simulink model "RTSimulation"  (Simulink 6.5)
settings: Solver=FixedStepDiscrete  StartTime=0.0  StopTime=inf  RelTol=1e-3
PreLoadFcn:
  | initialize
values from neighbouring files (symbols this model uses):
  actParams = [	bulkModulus   * pressCanon    [Copy of initialize.m]    (also in initialize.m = [bulkModulus	* pressCanon,)
  displFreq = inf    [initialize.m]
  flowCanon = 1.666667e+04    (= 16666.67)    [Copy of initialize.m]    (also in initialize.m)
  forceCanon = 1    [Copy of initialize.m]    (also in initialize.m)
  forceFreq = inf    [initialize.m]
  friction = 5			 				* 0.155000	 				* 0.00444822 				* area1    (= 2.71252900422)    [initialize.m]
  fsamp = 1 / samplePeriod    (= 1024)    [Copy of initialize.m]    (also in initialize.m; rampth.m = 1 / deltaT; randth.m = 1 / deltaT; rspect.m = 1.0 / tsamp)
  gasConstant = 1.8    [Copy of initialize.m]    (also in initialize.m)
  lengthCanon = 1    [Copy of initialize.m]    (also in initialize.m)
  massCanon = 1e-06    [Copy of initialize.m]    (also in initialize.m)
  maxDispl = ( (stroke2 + endLength2) * lengthCanon)'    [Copy of initialize.m]    (also in initialize.m = 576.2)
  maxOilVolume = volume * (1 - (precharge/supplyPress)^(1/gasConstant))    (= 211.391477114)    [Copy of initialize.m]    (also in initialize.m)
  maxVeloc = ( (maxFlow' * flowCanon ./ (area1 * areaCanon)) / velocCanon)'    [Copy of initialize.m]    (also in initialize.m = (maxFlow * flowCanon / (area1 * areaCanon)) / velocCanon; rampth.m = 2 * maxDispl / (nVeloc * deltaT))
  minDispl = (-(stroke1 + endLength1) * lengthCanon)'    [Copy of initialize.m]    (also in initialize.m = -576.2)
  minVeloc = (-(maxFlow' * flowCanon ./ (area2 * areaCanon)) / velocCanon)'    [Copy of initialize.m]    (also in initialize.m = -(maxFlow * flowCanon / (area2 * areaCanon)) / velocCanon)
  nAct = 5    [Copy of initialize.m]    (also in initialize.m = 1)
  nAdcU = 6    [Copy of initialize.m]    (also in initialize.m = 5)
  nDout = 4    [Copy of initialize.m]    (also in initialize.m)
  nDucU = 2    [Copy of initialize.m]    (also in initialize.m)
  nEncU = 3    [Copy of initialize.m]    (also in initialize.m)
  node = completenodestruct(node)    [Copy of initialize.m]    (also in initialize.m)
  precharge = 3000		 				* 6.894757e-03    (= 20.684271)    [Copy of initialize.m]    (also in initialize.m)
  pumpFlow = 1e20    (= 1e+20)    [Copy of initialize.m]    (also in initialize.m)
  returnPress = 3			 				* 0.1    (= 0.3)    [Copy of initialize.m]    (also in initialize.m)
  samplePeriod = controlPeriod/upsampleFactor    (= 0.0009765625)    [Copy of initialize.m]    (also in initialize.m; viewer.m = eval(getHeaderValue(header, 'DELTA_T')))
  springCanon = 1    [Copy of initialize.m]    (also in initialize.m)
  supplyPress = 280		 				* 0.1    (= 28)    [Copy of initialize.m]    (also in initialize.m)
  velocCanon = 1    [Copy of initialize.m]    (also in initialize.m)
  volume = 15.15		 				+ (  45		 				    * 2		 				   + 30		 				    * 6 )	 				* 5    (= 1365.15)    [Copy of initialize.m]    (also in initialize.m; quake.m = volume / 231.0)
  volumeCanon = 1e+06    (= 1000000)    [Copy of initialize.m]    (also in initialize.m)
  yieldDispl = 1.0    (= 1)    [initialize.m]
undefined symbols (not defined in the file or in its folder): DiscIntNeverNeededParam, dpforceFreq, mass, spring, staticForce
libraries: xpclib x5
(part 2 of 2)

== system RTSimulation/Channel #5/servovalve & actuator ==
  note: Parameter vector: 1: oil bulk modulus (force/displ^2) 2: servovalve delay (sec) 3: servovalve overlap 4: rated pressure (force/displ^2) 5: rated flow at rated pressure (displ^3/sec) 6: nominal flow at rated pressure (displ^3/sec) 7: actuator piston area 1 (displ^2) 8: actuator piston area 2 (displ^2) 9: actuator usable stroke 1 (displ) 10: actuator usable stroke 2 (displ) 11: actuator end cushion length 1 (displ) 12: actuator end cushion length 2 (displ) 13: additional port volume 1 (displ^3) 14: additional port volume 1 (displ^3) 15: actuator parasitic damping factor 16: cross-chamber leakage factor (flow/press) 17: ratio port openings according to area 18: sample period (sec) Conversion factors used for converting signals from external (user) to internal (canonical) units: 19: displacement 20: velocity 21: force 22: pressure 23: flow
  note: Note: "1" and "2" denote actuator cylinders on either side of the actuator piston. With positive valve drive, oil is ported into cylinder 1, resulting in positive displacement.
  note: Auxiliary diagnostic output vector: 1: valve opening 2: C1 pressure 3: C2 pressure 4: delta pressure 5: force 6: velocity 7: C1 flow 8: C2 flow 9: total flow 10: kinematic flow 11: compressibility flow 12: leakage flow 13: C1 oilspring displacement 14: C2 oilspring displacement 15: C1 oilspring velocity 16: C2 oilspring velocity
  cmd : Inport
  displ : Inport  Port=2
  veloc : Inport  Port=3
  spl press : Inport  Port=4
  rtn press : Inport  Port=5
  abs : Abs  SaturateOnIntegerOverflow=on  SampleTime=-1
  actuator : S-Function  FunctionName=Actuator  Parameters=params
  total flow sel : Selector  InputType=Vector  ElementSrc=Internal  Elements=9  RowSrc=Internal  Rows=1  ColumnSrc=Internal  Columns=1  IndexIsStartValue=off
  force : Outport
  flow : Outport  Port=2
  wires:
  spl press/1 -> actuator/4
  rtn press/1 -> actuator/5
  cmd/1 -> actuator/1
  actuator/1 -> force/1
  displ/1 -> actuator/2
  veloc/1 -> actuator/3
  actuator/2 -> total flow sel/1
  total flow sel/1 -> abs/1
  abs/1 -> flow/1

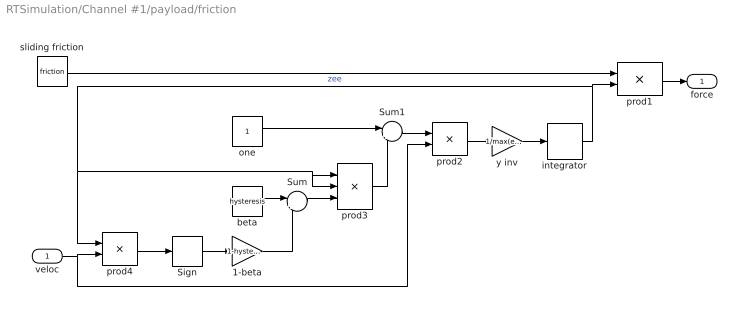
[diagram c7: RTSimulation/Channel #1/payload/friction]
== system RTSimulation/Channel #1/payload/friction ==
  veloc : Inport
  1-beta : Gain  Gain=1-hysteresis
  Sign : Signum
  Sum : Sum  Inputs=|++
  Sum1 : Sum  Inputs=|+-
  beta : Constant  Value=hysteresis  OutDataType=sfix(16)  ConRadixGroup=Use specified scaling  OutScaling=2^0  SampleTime=inf  FramePeriod=inf
  integrator : DiscreteIntegrator  SampleTime=-1  LimitOutput=on  UpperSaturationLimit=1  LowerSaturationLimit=-1  ICPrevOutput=DiscIntNeverNeededParam  ICPrevScaledInput=DiscIntNeverNeededParam
  one : Constant  Value=1  OutDataType=sfix(16)  ConRadixGroup=Use specified scaling  OutScaling=2^0  SampleTime=inf  FramePeriod=inf
  prod1 : Product
  prod2 : Product
  prod3 : Product  Inputs=3
  prod4 : Product
  sliding friction : Constant  Value=friction  OutDataType=sfix(16)  ConRadixGroup=Use specified scaling  OutScaling=2^0  SampleTime=inf  FramePeriod=inf
  y inv : Gain  Gain=1/max(eps, yieldDispl)
  force : Outport
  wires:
  integrator/1 -> prod3/2, prod3/1, prod4/1, prod1/2  "zee"
  y inv/1 -> integrator/1
  prod2/1 -> y inv/1
  Sum1/1 -> prod2/1
  prod3/1 -> Sum1/2
  one/1 -> Sum1/1
  Sum/1 -> prod3/3
  beta/1 -> Sum/1
  1-beta/1 -> Sum/2
  Sign/1 -> 1-beta/1
  prod4/1 -> Sign/1
  veloc/1 -> prod2/2, prod4/2
  prod1/1 -> force/1
  sliding friction/1 -> prod1/1

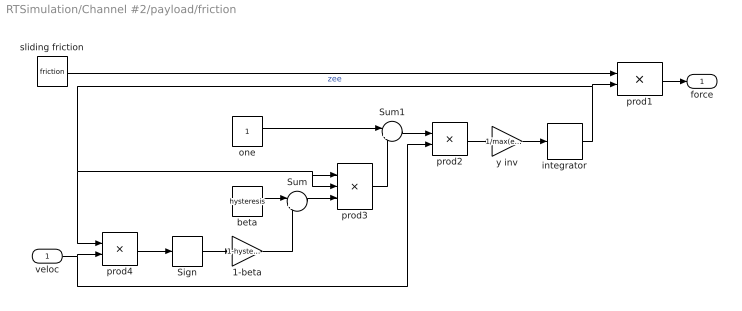
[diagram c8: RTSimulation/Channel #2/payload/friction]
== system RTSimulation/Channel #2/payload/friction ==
  veloc : Inport
  1-beta : Gain  Gain=1-hysteresis
  Sign : Signum
  Sum : Sum  Inputs=|++
  Sum1 : Sum  Inputs=|+-
  beta : Constant  Value=hysteresis  OutDataType=sfix(16)  ConRadixGroup=Use specified scaling  OutScaling=2^0  SampleTime=inf  FramePeriod=inf
  integrator : DiscreteIntegrator  SampleTime=-1  LimitOutput=on  UpperSaturationLimit=1  LowerSaturationLimit=-1  ICPrevOutput=DiscIntNeverNeededParam  ICPrevScaledInput=DiscIntNeverNeededParam
  one : Constant  Value=1  OutDataType=sfix(16)  ConRadixGroup=Use specified scaling  OutScaling=2^0  SampleTime=inf  FramePeriod=inf
  prod1 : Product
  prod2 : Product
  prod3 : Product  Inputs=3
  prod4 : Product
  sliding friction : Constant  Value=friction  OutDataType=sfix(16)  ConRadixGroup=Use specified scaling  OutScaling=2^0  SampleTime=inf  FramePeriod=inf
  y inv : Gain  Gain=1/max(eps, yieldDispl)
  force : Outport
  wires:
  sliding friction/1 -> prod1/1
  prod1/1 -> force/1
  veloc/1 -> prod4/2, prod2/2
  prod4/1 -> Sign/1
  Sign/1 -> 1-beta/1
  1-beta/1 -> Sum/2
  beta/1 -> Sum/1
  Sum/1 -> prod3/3
  one/1 -> Sum1/1
  prod3/1 -> Sum1/2
  Sum1/1 -> prod2/1
  prod2/1 -> y inv/1
  y inv/1 -> integrator/1
  integrator/1 -> prod1/2, prod4/1, prod3/1, prod3/2  "zee"

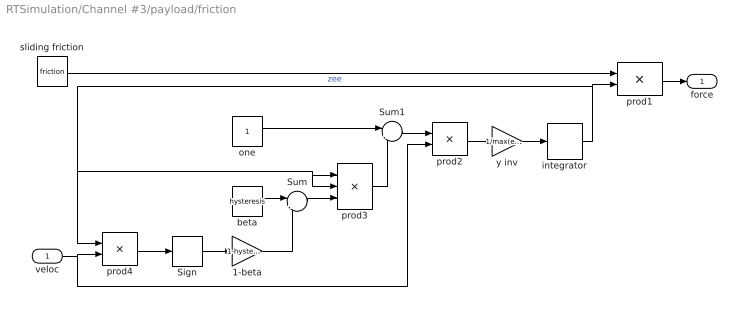
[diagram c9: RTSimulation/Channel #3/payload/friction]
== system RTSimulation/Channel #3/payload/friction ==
  veloc : Inport
  1-beta : Gain  Gain=1-hysteresis
  Sign : Signum
  Sum : Sum  Inputs=|++
  Sum1 : Sum  Inputs=|+-
  beta : Constant  Value=hysteresis  OutDataType=sfix(16)  ConRadixGroup=Use specified scaling  OutScaling=2^0  SampleTime=inf  FramePeriod=inf
  integrator : DiscreteIntegrator  SampleTime=-1  LimitOutput=on  UpperSaturationLimit=1  LowerSaturationLimit=-1  ICPrevOutput=DiscIntNeverNeededParam  ICPrevScaledInput=DiscIntNeverNeededParam
  one : Constant  Value=1  OutDataType=sfix(16)  ConRadixGroup=Use specified scaling  OutScaling=2^0  SampleTime=inf  FramePeriod=inf
  prod1 : Product
  prod2 : Product
  prod3 : Product  Inputs=3
  prod4 : Product
  sliding friction : Constant  Value=friction  OutDataType=sfix(16)  ConRadixGroup=Use specified scaling  OutScaling=2^0  SampleTime=inf  FramePeriod=inf
  y inv : Gain  Gain=1/max(eps, yieldDispl)
  force : Outport
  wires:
  integrator/1 -> prod3/2, prod3/1, prod4/1, prod1/2  "zee"
  y inv/1 -> integrator/1
  prod2/1 -> y inv/1
  Sum1/1 -> prod2/1
  prod3/1 -> Sum1/2
  one/1 -> Sum1/1
  Sum/1 -> prod3/3
  beta/1 -> Sum/1
  1-beta/1 -> Sum/2
  Sign/1 -> 1-beta/1
  prod4/1 -> Sign/1
  veloc/1 -> prod2/2, prod4/2
  prod1/1 -> force/1
  sliding friction/1 -> prod1/1

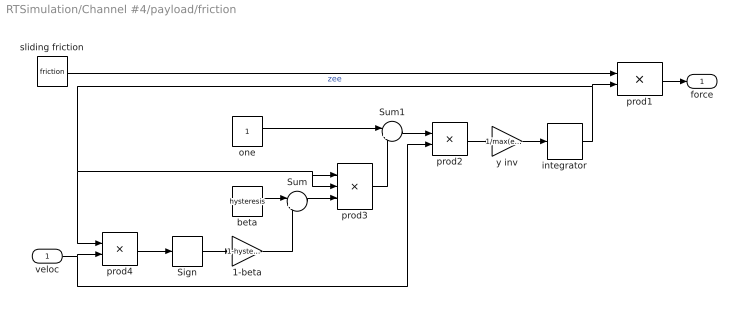
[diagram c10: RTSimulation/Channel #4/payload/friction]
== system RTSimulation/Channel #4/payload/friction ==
  veloc : Inport
  1-beta : Gain  Gain=1-hysteresis
  Sign : Signum
  Sum : Sum  Inputs=|++
  Sum1 : Sum  Inputs=|+-
  beta : Constant  Value=hysteresis  OutDataType=sfix(16)  ConRadixGroup=Use specified scaling  OutScaling=2^0  SampleTime=inf  FramePeriod=inf
  integrator : DiscreteIntegrator  SampleTime=-1  LimitOutput=on  UpperSaturationLimit=1  LowerSaturationLimit=-1  ICPrevOutput=DiscIntNeverNeededParam  ICPrevScaledInput=DiscIntNeverNeededParam
  one : Constant  Value=1  OutDataType=sfix(16)  ConRadixGroup=Use specified scaling  OutScaling=2^0  SampleTime=inf  FramePeriod=inf
  prod1 : Product
  prod2 : Product
  prod3 : Product  Inputs=3
  prod4 : Product
  sliding friction : Constant  Value=friction  OutDataType=sfix(16)  ConRadixGroup=Use specified scaling  OutScaling=2^0  SampleTime=inf  FramePeriod=inf
  y inv : Gain  Gain=1/max(eps, yieldDispl)
  force : Outport
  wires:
  sliding friction/1 -> prod1/1
  prod1/1 -> force/1
  veloc/1 -> prod4/2, prod2/2
  prod4/1 -> Sign/1
  Sign/1 -> 1-beta/1
  1-beta/1 -> Sum/2
  beta/1 -> Sum/1
  Sum/1 -> prod3/3
  one/1 -> Sum1/1
  prod3/1 -> Sum1/2
  Sum1/1 -> prod2/1
  prod2/1 -> y inv/1
  y inv/1 -> integrator/1
  integrator/1 -> prod1/2, prod4/1, prod3/1, prod3/2  "zee"

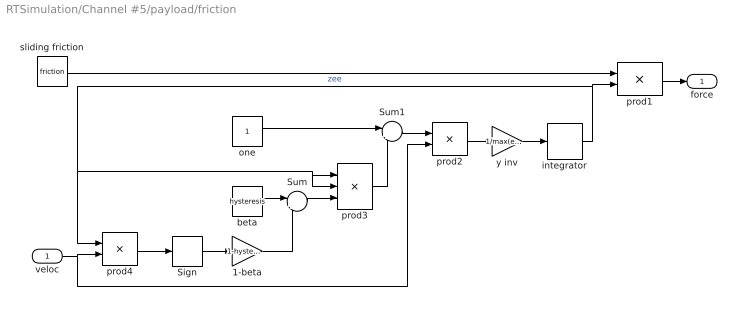
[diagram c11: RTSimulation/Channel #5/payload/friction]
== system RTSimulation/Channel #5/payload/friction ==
  veloc : Inport
  1-beta : Gain  Gain=1-hysteresis
  Sign : Signum
  Sum : Sum  Inputs=|++
  Sum1 : Sum  Inputs=|+-
  beta : Constant  Value=hysteresis  OutDataType=sfix(16)  ConRadixGroup=Use specified scaling  OutScaling=2^0  SampleTime=inf  FramePeriod=inf
  integrator : DiscreteIntegrator  SampleTime=-1  LimitOutput=on  UpperSaturationLimit=1  LowerSaturationLimit=-1  ICPrevOutput=DiscIntNeverNeededParam  ICPrevScaledInput=DiscIntNeverNeededParam
  one : Constant  Value=1  OutDataType=sfix(16)  ConRadixGroup=Use specified scaling  OutScaling=2^0  SampleTime=inf  FramePeriod=inf
  prod1 : Product
  prod2 : Product
  prod3 : Product  Inputs=3
  prod4 : Product
  sliding friction : Constant  Value=friction  OutDataType=sfix(16)  ConRadixGroup=Use specified scaling  OutScaling=2^0  SampleTime=inf  FramePeriod=inf
  y inv : Gain  Gain=1/max(eps, yieldDispl)
  force : Outport
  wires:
  integrator/1 -> prod3/2, prod3/1, prod4/1, prod1/2  "zee"
  y inv/1 -> integrator/1
  prod2/1 -> y inv/1
  Sum1/1 -> prod2/1
  prod3/1 -> Sum1/2
  one/1 -> Sum1/1
  Sum/1 -> prod3/3
  beta/1 -> Sum/1
  1-beta/1 -> Sum/2
  Sign/1 -> 1-beta/1
  prod4/1 -> Sign/1
  veloc/1 -> prod2/2, prod4/2
  prod1/1 -> force/1
  sliding friction/1 -> prod1/1
